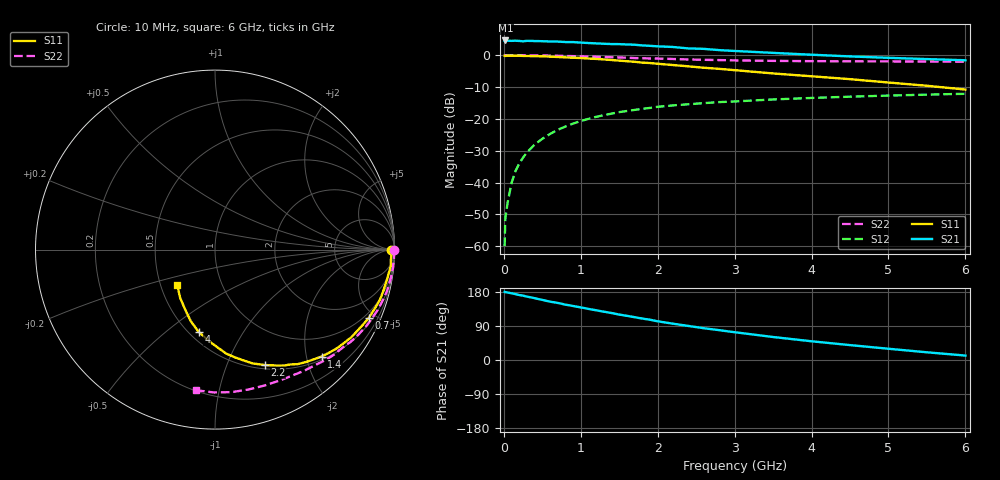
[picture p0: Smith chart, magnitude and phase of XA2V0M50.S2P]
! SIEMENS Discrete & RF Semiconductors
! BFY180
! Si NPN RF Bipolar Junction Transistor in MICRO-X
! VCE = 2 V  IC = 0.5 mA
! Common Emitter S-Parameters:  May  1997
# GHz  S  MA  R  50
!  f  S11  S21  S12  S22
! GHz  MAG  ANG  MAG  ANG  MAG  ANG  MAG  ANG
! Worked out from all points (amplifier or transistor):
!   36 points, 10 MHz to 6 GHz, reference 50 ohm
!   highest |S21| = 4.6 dB at 20 MHz (marker M1)
!   |S21| within 3 dB of that: start of sweep to 2.782 GHz
!   unconditionally stable (mu >= 1): 5.145 GHz to end of sweep
!   at 250 MHz: K = 0.05, MSG = 18.3 dB, |S12| = -32.1 dB
!   at 1.4 GHz: K = 0.41, MSG = 10.9 dB, |S12| = -18.4 dB
!   at 6 GHz: K = 1.03, MAG = 4.2 dB, |S12| = -12.1 dB
!   S11 on the Smith chart (normalised r, x): 10 MHz: 90, -14; 700 MHz: 0.73, -4.61; 1.4 GHz: 0.56, -2.29; 2.2 GHz: 0.54, -1.37; 4 GHz: 0.56, -0.65; 6 GHz: 0.61, -0.26
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0.01  0.9785 -0.2  1.667 179.9  0.001 81.6  0.9992 -0.2
0.02  0.9735 -0.8  1.705 179.0  0.0028 87.0  0.9999 -0.5
0.05  0.9838 -1.7  1.687 178.1  0.0049 86.4  0.9986 -1.1
0.1  0.9811 -3.4  1.68 176.0  0.0098 87.3  0.9982 -2.3
0.15  0.9836 -5.3  1.689 173.9  0.015 86.6  0.9984 -3.5
0.2  0.9795 -6.8  1.676 171.5  0.0198 85.7  0.9962 -4.6
0.3  0.9719 -10.2  1.682 167.3  0.0296 82.2  0.9943 -6.9
0.4  0.9662 -13.5  1.67 163.1  0.0395 79.7  0.9927 -9.2
0.6  0.9495 -20.1  1.644 154.0  0.0579 74.5  0.9852 -13.7
0.7  0.9378 -23.9  1.636 150.7  0.0672 71.5  0.9791 -15.9
0.9  0.9132 -29.7  1.609 142.6  0.0843 66.6  0.9664 -20.4
1.1  0.8871 -36.0  1.554 134.9  0.0999 61.8  0.9517 -24.5
1.4  0.841 -45.1  1.497 124.0  0.1209 55.1  0.929 -30.6
1.7  0.7877 -54.1  1.461 113.0  0.1383 49.0  0.9022 -36.2
2.2  0.7003 -66.7  1.346 95.8  0.1627 40.1  0.8717 -44.8
2.6  0.6358 -75.8  1.258 83.9  0.1767 34.5  0.8465 -50.7
3  0.5824 -83.9  1.166 73.3  0.1878 29.1  0.8287 -56.5
3.5  0.517 -92.8  1.088 60.7  0.2018 23.8  0.8148 -63.1
4  0.4667 -101.3  1.018 49.4  0.2131 18.4  0.8062 -69.8
4.5  0.4205 -108.8  0.957 39.3  0.2232 13.7  0.8015 -76.5
5.5  0.331 -126.0  0.869 20.3  0.2403 4.5  0.7958 -90.5
6  0.2888 -136.5  0.833 11.7  0.2476 -0.2  0.7904 -97.6
